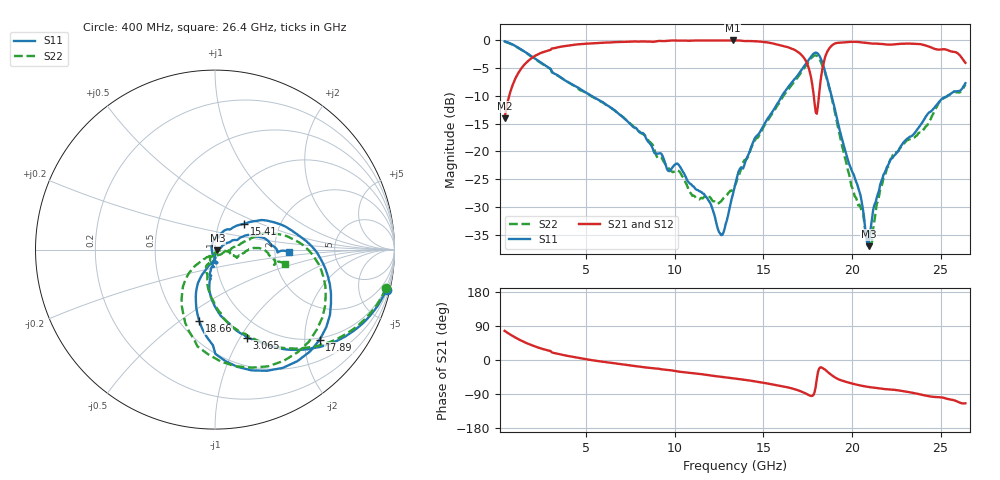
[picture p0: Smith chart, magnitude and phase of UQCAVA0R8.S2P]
!  Part Number  UQCQVA0R8	Mounting Orientation: Horizontal
!  Description: RF capacitors
!  Application: Coupling, Bypass, Tuning, DC Block
!  Filters, Matching
# GHZ S DB R 50
! Freq  |S11|  S11 Ph  |S21|  S21 Ph  |S12|  S12 Ph  |S22|  S22 Ph
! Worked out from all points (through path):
!   401 points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, 400 MHz to 26.4 GHz, reference 50 ohm
!   highest |S21| = 0.00 dB at 13.27 GHz (marker M1); lowest = -14.0 dB at 400 MHz (marker M2)
!   group delay of S21, straight-line fit = 15.1 ps
!   lowest |S11| = -37.1 dB at 20.94 GHz (marker M3), VSWR 1.03, Z = 51.3 - j0.505 ohm
!   |S11| at or under -10 dB: 5.308 GHz to 16.05 GHz (10.74 GHz wide, 101 % of centre); 18.85 GHz to 25.4 GHz (6.555 GHz wide, 29.6 % of centre)
!   |S22| runs from -36.8 to -0.2 dB; largest |S21 - S12| = 0.0084
!   S11 on the Smith chart (normalised r, x): 400 MHz: 0.70, -8.65; 3.065 GHz: 0.79, -1.07; 15.41 GHz: 1.32, +0.40; 17.89 GHz: 0.95, -2.36; 18.66 GHz: 0.62, -0.60; 26.4 GHz: 2.40, -0.07
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0.4  -0.16 -13.1  -14.03 76.8  -14.03 76.8  -0.21 -12.7
1.31  -1.58 -38.5  -5.19 51.8  -5.20 51.8  -1.61 -37.7
3.065  -5.64 -70.0  -1.44 20.0  -1.45 20.1  -5.74 -69.0
4.755  -8.94 -86.1  -0.65 3.9  -0.65 3.9  -9.06 -85.2
9.11  -20.38 -93.1  -0.08 -23.3  -0.06 -23.2  -21.30 -111.3
11.775  -28.24 -95.8  -0.01 -39.2  -0.01 -39.2  -28.14 -89.5
12.62  -35.10 -164.7  -0.01 -44.3  -0.01 -44.3  -29.00 -58.1
13.27  -27.89 109.7  0.00 -48.2  -0.01 -48.3  -26.97 -28.7
13.4  -26.05 100.9  -0.01 -49.0  -0.01 -49.0  -26.12 -18.8
15.415  -13.28 41.8  -0.46 -63.7  -0.44 -63.8  -13.58 17.4
16.975  -6.14 7.3  -2.12 -80.2  -2.10 -80.4  -6.47 4.5
17.755  -2.65 -29.7  -7.85 -94.7  -7.82 -95.0  -3.00 -32.3
17.885  -2.27 -40.8  -11.18 -86.1  -11.14 -86.2  -2.70 -44.4
18.21  -3.06 -73.2  -7.77 -19.5  -7.74 -19.7  -3.62 -80.2
18.665  -7.76 -102.3  -1.69 -33.0  -1.67 -33.3  -7.94 -116.2
19.315  -16.29 -117.0  -0.40 -52.4  -0.38 -52.7  -17.16 -140.9
20.42  -27.23 -90.8  -0.30 -66.7  -0.28 -67.0  -29.59 -110.2
20.94  -37.10 -20.6  -0.48 -71.3  -0.46 -71.6  -35.95 -71.0
21.33  -29.22 18.1  -0.57 -73.5  -0.56 -73.7  -31.19 -11.8
22.11  -22.00 28.4  -0.77 -77.7  -0.75 -78.0  -21.90 -10.8
23.93  -14.97 24.9  -0.71 -91.7  -0.69 -92.1  -16.34 -10.2
26.4  -7.70 -1.8  -4.03 -114.2  -4.02 -114.7  -7.98 -11.3
